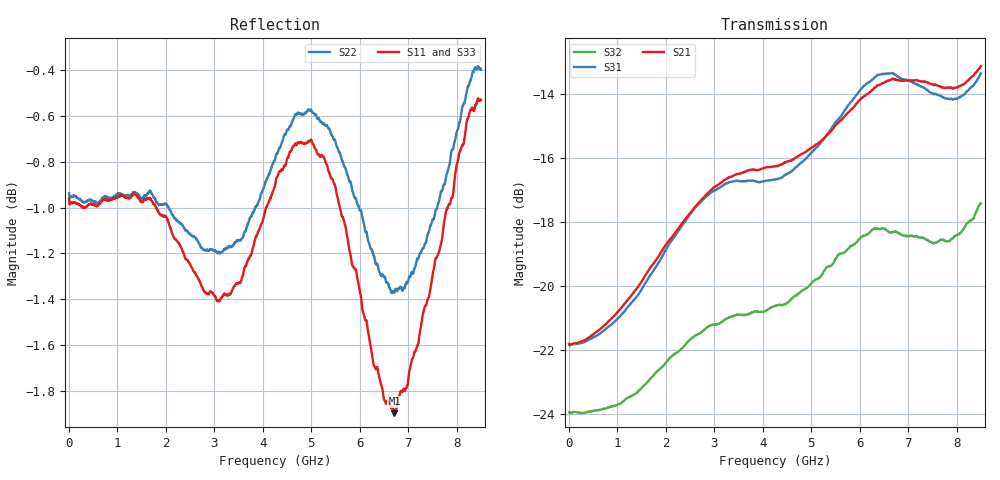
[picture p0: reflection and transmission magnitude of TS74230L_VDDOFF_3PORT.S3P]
!Agilent Technologies,E5071C,MY46522130,B.12.04
!Date: Wed Jul 30 10:24:27 2025
!Data & Calibration Information:
!Freq	S11:SOLT3(ON)	S13:SOLT3(ON)	S14:SOLT3(ON)
!	S31:SOLT3(ON)	S33:SOLT3(ON)	S34:SOLT3(ON)
!	S41:SOLT3(ON)	S43:SOLT3(ON)	S44:SOLT3(ON)
!PortZ  Port1:50+j0  Port3:50+j0  Port4:50+j0
!Above PortZ is port z conversion or system Z0 setting when saving the data.
!When reading, reference impedance value at option line is always used.
# Hz S dB R 50
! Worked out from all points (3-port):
!   1601 points, 10 MHz to 8.5 GHz, reference 50 ohm
!   strongest paths, dB at 10 MHz, 2.132 GHz, 4.255 GHz, 6.378 GHz, 8.5 GHz:
!     S21: -21.8, -18.5, -16.3, -13.7, -13.1
!     S31: -21.8, -18.6, -16.7, -13.4, -13.4
!     S32: -24.0, -22.2, -20.6, -18.2, -17.4
!   lowest |S11| = -1.9 dB at 6.717 GHz (marker M1), VSWR 9.19, Z = 18.2 + j75.1 ohm
!   |S11| at or under -10 dB: nowhere
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1e7  -0.96 179.4  -21.82 -0.4  -21.83 -0.4
     -21.82 -0.4  -0.94 179.4  -23.95 -0.5
     -21.82 -0.4  -23.95 -0.6  -0.93 179.4
9.22675e8  -0.96 161.0  -20.96 8.5  -21.15 7.8
           -20.96 8.5  -0.95 159.7  -23.78 -0.4
           -21.16 7.7  -23.76 -0.3  -0.94 160.3
2.015762e9  -1.04 144.8  -18.69 8.8  -18.84 9.2
            -18.69 8.7  -0.99 138.9  -22.37 -2.9
            -18.84 9.1  -22.39 -3.0  -1.01 141.4
3.61825e9  -1.27 106.8  -16.44 -9.5  -16.72 -11.2
           -16.44 -9.6  -1.11 106.0  -20.93 -20.8
           -16.73 -11.2  -20.91 -21.0  -1.09 103.2
4.255e9  -0.90 98.0  -16.28 -15.9  -16.69 -16.1
         -16.28 -16.1  -0.79 95.1  -20.69 -26.8
         -16.69 -16.2  -20.63 -26.5  -0.75 95.6
5.624012e9  -1.03 92.1  -14.80 -25.6  -14.67 -24.7
            -14.83 -25.6  -0.79 82.9  -19.06 -38.4
            -14.69 -24.7  -19.00 -38.4  -0.88 85.2
6.7171e9  -1.90 65.2  -13.55 -43.7  -13.38 -46.9
          -13.56 -44.0  -1.37 65.4  -18.34 -58.5
          -13.40 -47.3  -18.32 -58.2  -1.50 57.7
7.555488e9  -1.23 46.9  -13.69 -54.8  -14.01 -57.6
            -13.71 -55.2  -1.02 50.4  -18.53 -65.4
            -14.00 -57.7  -18.65 -65.8  -0.93 45.4
8.001212e9  -0.81 44.9  -13.81 -58.7  -14.12 -60.2
            -13.80 -59.0  -0.67 45.5  -18.50 -68.5
            -14.15 -60.2  -18.42 -68.5  -0.60 43.5
8.5e9  -0.53 49.2  -13.13 -60.7  -13.35 -60.0
       -13.14 -60.9  -0.40 44.3  -17.47 -71.5
       -13.36 -60.3  -17.43 -70.5  -0.38 46.1
